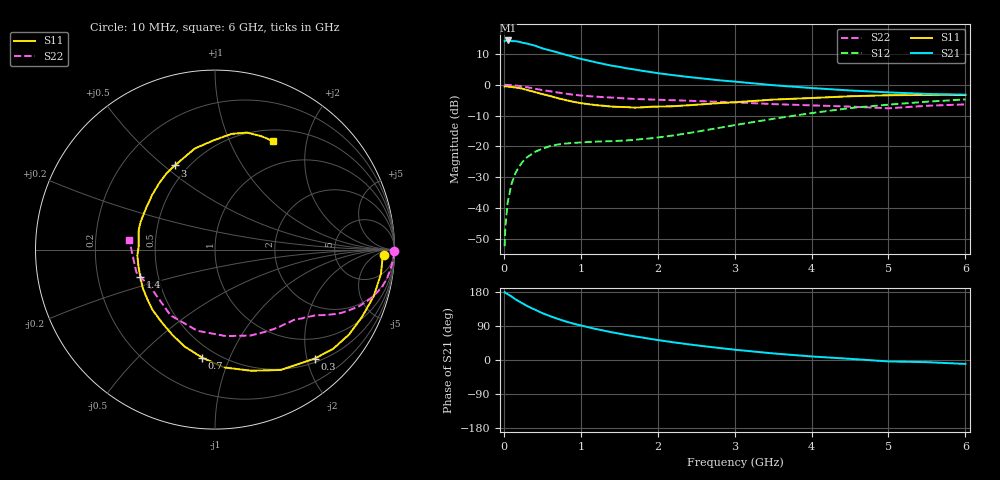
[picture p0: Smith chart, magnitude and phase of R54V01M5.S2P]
! SIEMENS Small Signal Semiconductors
! BFR183
! Si NPN RF Bipolar Junction Transistor in SOT23
! VCE = 4 V  IC = 1.5 mA
! Common Emitter S-Parameters:  May  1996
# GHz  S  MA  R  50
!  f  S11  S21  S12  S22
! GHz  MAG  ANG  MAG  ANG  MAG  ANG  MAG  ANG
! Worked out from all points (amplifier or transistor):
!   36 points, 10 MHz to 6 GHz, reference 50 ohm
!   highest |S21| = 14.4 dB at 50 MHz (marker M1)
!   |S21| within 3 dB of that: start of sweep to 565.4 MHz
!   unconditionally stable (mu >= 1): 1.528 GHz to 2.882 GHz
!   at 250 MHz: K = 0.19, MSG = 19.2 dB, |S12| = -24.8 dB
!   at 1.4 GHz: K = 0.95, MSG = 12.3 dB, |S12| = -18.3 dB
!   at 6 GHz: K = 0.92, MSG = 0.8 dB, |S12| = -4.8 dB
!   S11 on the Smith chart (normalised r, x): 10 MHz: 26, -12; 300 MHz: 0.57, -2.15; 700 MHz: 0.42, -0.80; 1.4 GHz: 0.40, -0.15; 3 GHz: 0.42, +0.55; 6 GHz: 0.64, +1.46
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0.01  0.9392 -1.7  5.103 179.1  0.0024 92.5  0.9974 -0.6
0.02  0.9346 -3.2  5.188 177.3  0.0049 80.1  0.9966 -1.3
0.05  0.9345 -8.4  5.238 173.7  0.0124 84.7  0.9949 -3.2
0.1  0.9215 -16.4  5.114 167.6  0.0246 80.7  0.9838 -6.3
0.15  0.9011 -24.6  5.096 160.3  0.0367 75.4  0.9724 -9.4
0.2  0.8839 -32.4  4.978 154.4  0.0472 71.4  0.956 -12.2
0.3  0.8231 -47.5  4.653 142.7  0.0662 63.7  0.9136 -17.1
0.4  0.7645 -61.3  4.336 133.2  0.0809 56.7  0.8649 -21.3
0.5  0.7047 -73.3  3.901 123.7  0.0917 51.7  0.8196 -24.4
0.6  0.6584 -85.6  3.61 115.9  0.1009 47.2  0.7845 -26.8
0.7  0.606 -96.8  3.351 108.6  0.1071 44.1  0.7497 -28.7
0.8  0.5655 -107.6  3.081 102.0  0.111 41.3  0.7186 -30.5
0.9  0.5304 -116.7  2.845 96.2  0.1139 39.7  0.6907 -31.9
1.1  0.4844 -135.7  2.468 86.4  0.1179 38.1  0.6541 -34.5
1.4  0.4428 -160.0  2.044 73.3  0.1214 38.4  0.6195 -38.2
1.7  0.4252 177.6  1.769 62.5  0.1277 43.0  0.5877 -41.8
2.2  0.4483 148.8  1.434 46.8  0.1503 50.4  0.5615 -49.7
3  0.5197 115.5  1.126 27.2  0.2214 55.5  0.5183 -67.5
3.5  0.5743 101.3  0.984 17.4  0.2798 52.8  0.4858 -82.8
4.5  0.6508 82.0  0.808 3.1  0.4184 40.9  0.4423 -124.1
5.5  0.6829 67.6  0.71 -5.7  0.5311 25.3  0.456 -163.9
6  0.6846 62.0  0.69 -10.4  0.5779 15.7  0.4798 173.9
